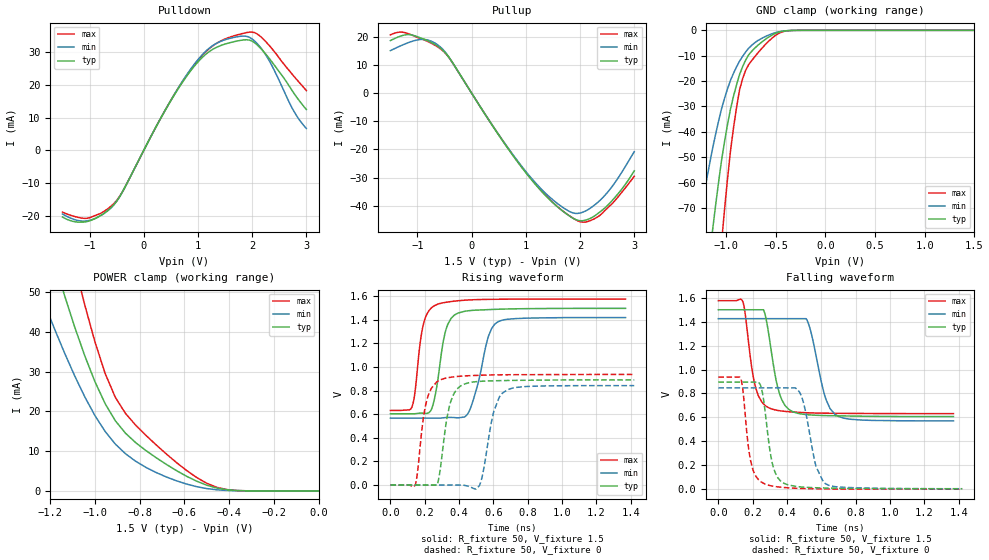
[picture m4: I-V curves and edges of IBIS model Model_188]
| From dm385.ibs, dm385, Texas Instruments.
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| Model based on original model for BCSHTLTCSCDVPBFZ_SSDHV
|   Sub model SR00_11MA_5PER_1P5
[model]   Model_188
|[Description]  [1.5V-3-STATE-NOTERM-FASTEST:11MA, IND, 5%]
|   Fastest slew rate (SR[1:0] = "00"), 0.73 * RExt = 1.325 * Iout
|   (I[2:0] = "110"), 11mA nominal with Rext = 50R,ODT off (ODT[1:0]
|   = "00") CMOS mode,Industrial temperature range (-40C to 125C,
|   25C nominal),5% power supply tolerance
|[Input Load]   NOTERM
|[Output Drive] FASTEST:11MA
|Voltage   1.5V
|Mode   3-STATE
Model_type   3-state
Polarity   Non-Inverting
Enable   Active-Low
Cref =  15pF
Rref =  100.0000M
Vref =  0V
Vmeas =  0.75
C_comp   1.865048p   1.679967p   1.989968p
[Temperature Range]   25   125   -40
[Voltage Range]   1.5   1.425   1.575
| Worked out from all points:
|   slope of the pulldown table from 0 to 0.225 V, typ, clamps not added: 31.7 ohm
|   slope of the pullup table from 0 to 0.225 V, typ, clamps not added: 32.8 ohm
|   GND clamp passes 1 mA (typ) near -0.49 V on its own axis
|   POWER clamp passes 1 mA (typ) near -0.47 V on its own axis
|   rising waveform, R_fixture 50, V_fixture 1.5: 20-80 % time 59.9ps typ, 82.4ps min, 51ps max; typ from 0.603 V to 1.5 V
|   rising waveform, R_fixture 50, V_fixture 0: 20-80 % time 58.5ps typ, 68ps min, 54.4ps max; typ from 0 V to 0.89 V
|   falling waveform, R_fixture 50, V_fixture 1.5: 20-80 % time 68.6ps typ, 80.3ps min, 60.7ps max; typ from 1.5 V to 0.607 V
|   falling waveform, R_fixture 50, V_fixture 0: 20-80 % time 54.2ps typ, 71.3ps min, 48.3ps max; typ from 0.895 V to 0.004 V
[POWER_clamp]
-1.5V     126mA      88.76mA    168.8mA
-1.242V   69.8mA     49.43mA    94.36mA
-1.136V   49.16mA    34.7mA     67.53mA
-1.061V   36.35mA    25.39mA    50.04mA
-1.045V   33.92mA    23.62mA    46.67mA
-954.5mV  21.93mA    14.94mA    29.52mA
-909.1mV  17.64mA    11.78mA    23.53mA
-863.6mV  14.51mA    9.346mA    19.48mA
-772.7mV  10.16mA    5.937mA    14mA
-590.9mV  3.705mA    1.741mA    5.168mA
-454.5mV  710.5uA    279.1uA    892.2uA
0V        1.424nA    14.75nA    2.169nA
[Pulldown]
-1.5V     -20.32mA   -19.41mA   -18.83mA
-1.045V   -21.71mA   -21.48mA   -20.72mA
-545.5mV  -16.46mA   -16.48mA   -16.11mA
-409.1mV  -13.12mA   -13.16mA   -13.06mA
727.3mV   21.07mA    21.41mA    21.29mA
1.136V    29.18mA    30.1mA     29.92mA
1.455V    32.16mA    33.45mA    33.62mA
1.864V    33.7mA     34.83mA    35.78mA
2.091V    32.17mA    32.59mA    35.5mA
2.318V    27.97mA    27.26mA    31.92mA
2.773V    17.36mA    11.84mA    22.54mA
3V        12.44mA    6.666mA    18.22mA
[Pullup]
-1.5V     18.7mA     15.13mA    20.75mA
-1.136V   20.8mA     18.2mA     20.93mA
-863.6mV  19.07mA    19.1mA     18.82mA
-590.9mV  16.22mA    16.64mA    15.97mA
-409.1mV  12.51mA    12.49mA    12.37mA
954.5mV   -27.15mA   -26.75mA   -27.01mA
1.409V    -37.28mA   -36.4mA    -37.19mA
1.818V    -43.8mA    -42.17mA   -43.78mA
2.045V    -45.32mA   -42.33mA   -45.84mA
2.318V    -42.92mA   -38.95mA   -44.05mA
2.636V    -37.2mA    -31.98mA   -38.33mA
3V        -27.6mA    -20.81mA   -29.54mA
[GND_clamp]
-1.5V     -219.3mA   -131.6mA   -364.3mA
-1.288V   -134.4mA   -79.74mA   -225.6mA
-1.258V   -122.9mA   -72.77mA   -206.3mA
-1.136V   -79.27mA   -46.88mA   -132.4mA
-1.045V   -51.5mA    -31.06mA   -84.11mA
-1.015V   -44.02mA   -26.9mA    -70.91mA
-954.5mV  -31.01mA   -19.7mA    -47.55mA
-863.6mV  -17.48mA   -12.16mA   -23.55mA
-803mV    -11.81mA   -8.597mA   -15.85mA
-681.8mV  -5.986mA   -4.096mA   -9.026mA
-378.8mV  -126.2uA   -131.8uA   -179.7uA
1.5V      1.424nA    36.56nA    1.506nA
[Ramp]
dV/dt_f 0.54961524/69.79814p  0.52871822/82.186467p 0.57471025/60.187411p
dV/dt_r 0.54896082/59.337024p 0.52750049/67.186701p 0.57134378/54.470647p
R_load = 50
[Rising Waveform]
R_fixture = 50
V_fixture = 1.5
V_fixture_min = 1.425
V_fixture_max = 1.575
0s        603.4mV    566.9mV    632.2mV
124.9ps   603.4mV    566.9mV    658mV
191.2ps   608mV      566.9mV    1.354V
264.2ps   782.6mV    566.9mV    1.524V
324.4ps   1.32V      571.7mV    1.548V
394.4ps   1.456V     569.1mV    1.561V
464.2ps   1.478V     641.7mV    1.568V
572.4ps   1.486V     1.266V     1.572V
631.1ps   1.489V     1.386V     1.573V
1.37ns    1.496V     1.418V     1.575V
[Rising Waveform]
R_fixture = 50
V_fixture = 0
V_fixture_min = 0
V_fixture_max = 0
0s        0V         0V         0V
145.5ps   0V         0V         2.162mV
209.8ps   0V         0V         705mV
290.8ps   135.9mV    0V         890.2mV
344.6ps   671.6mV    0V         911.3mV
423.3ps   850.8mV    0V         923.3mV
519.5ps   877.8mV    -3.609mV   929.5mV
602.5ps   882.9mV    624.5mV    932.6mV
684.3ps   885.5mV    808.6mV    934.1mV
1.421ns   890.2mV    841.9mV    936.7mV
[Falling Waveform]
R_fixture = 50
V_fixture = 1.5
V_fixture_min = 1.425
V_fixture_max = 1.575
0s        1.5V       1.425V     1.576V
139.5ps   1.5V       1.425V     1.579V
218ps     1.5V       1.425V     846.5mV
263.5ps   1.5V       1.425V     712mV
296.1ps   1.275V     1.425V     679.2mV
357.4ps   793.9mV    1.425V     655.6mV
435.3ps   646.8mV    1.425V     645mV
518.2ps   622.5mV    1.409V     638.6mV
679.1ps   613.5mV    626.4mV    634.1mV
1.37ns    607.1mV    571.1mV    631.4mV
[Falling Waveform]
R_fixture = 50
V_fixture = 0
V_fixture_min = 0
V_fixture_max = 0
0s        894.9mV    846.8mV    936.9mV
130.6ps   894.9mV    846.8mV    924.6mV
188.6ps   894.9mV    846.8mV    236mV
270.3ps   678.3mV    846.8mV    44.48mV
320.1ps   186.2mV    846.8mV    24.44mV
395.2ps   41.13mV    846.8mV    12.54mV
483.9ps   18.4mV     777.6mV    5.873mV
569.1ps   11.85mV    190mV      3.222mV
626ps     9.722mV    44.14mV    2.275mV
1.421ns   3.636mV    3.506mV    0V
